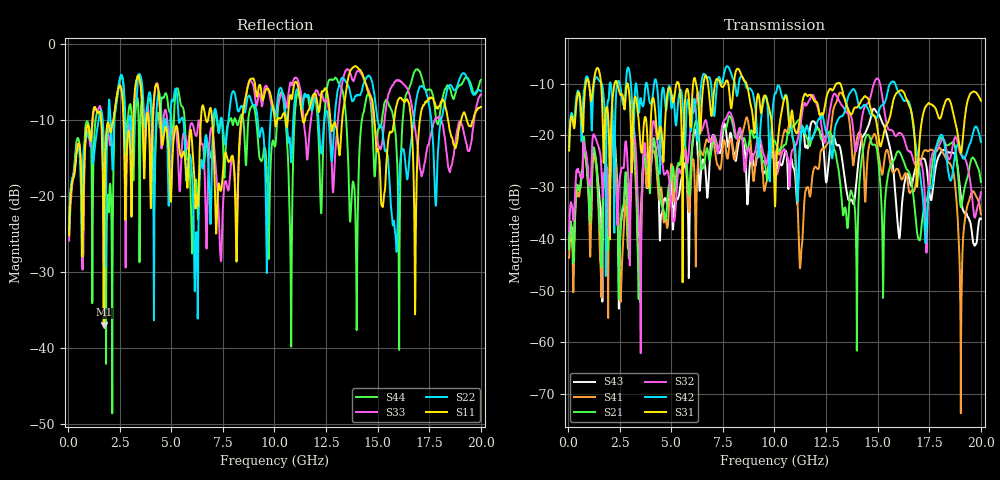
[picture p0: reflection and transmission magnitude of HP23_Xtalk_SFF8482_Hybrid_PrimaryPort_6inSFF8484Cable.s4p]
# MHz S MA R 50.00
! FREQ  S11  S12  S13  S14
!  S21  S22  S23  S24
!  S31  S32  S33  S34
!  S41  S42  S43  S44
!  MAG  ANG  MAG  ANG  MAG  ANG  MAG  ANG
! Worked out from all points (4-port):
!   1996 points, 50 MHz to 20 GHz, reference 50 ohm
!   strongest paths, dB at 50 MHz, 5.04 GHz, 10.03 GHz, 15.02 GHz, 20 GHz:
!     S31: -22.9, -12.7, -33.7, -19.6, -13.3
!     S42: -22.0, -13.9, -11.9, -15.8, -21.2
!     S32: -38.5, -35.4, -24.8, -9.1, -31.0
!     S21: -42.0, -26.6, -21.2, -24.5, -29.0
!     S41: -43.7, -26.5, -24.5, -23.0, -35.3
!     S43: -41.9, -32.6, -25.6, -15.7, -36.2
!   lowest |S11| = -36.9 dB at 1.73 GHz (marker M1), VSWR 1.03, Z = 48.8 + j0.648 ohm
!   |S11| at or under -10 dB: start of sweep to 1.177 GHz; 4.479 GHz to 6.435 GHz (1.956 GHz wide, 35.8 % of centre); 6.981 GHz to 8.398 GHz (1.417 GHz wide, 18.4 % of centre)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
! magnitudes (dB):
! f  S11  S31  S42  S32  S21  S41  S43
! 50 MHz  -25.2  -22.9  -22.0  -38.5  -42.0  -43.7  -41.9
! 1.73 GHz  -36.9  -25.3  -12.8  -27.3  -28.8  -28.5  -28.9
! 10.74 GHz  -7.0  -18.3  -17.2  -29.5  -18.9  -17.7  -26.4
! 11.27 GHz  -8.1  -15.6  -20.1  -17.6  -17.6  -44.6  -20.3
! 13.21 GHz  -12.7  -10.1  -16.4  -13.8  -30.2  -11.7  -22.9
! 15.87 GHz  -8.6  -12.1  -10.2  -20.1  -24.0  -26.7  -31.9
! 20 GHz  -8.3  -13.3  -21.2  -31.0  -29.0  -35.3  -36.2
